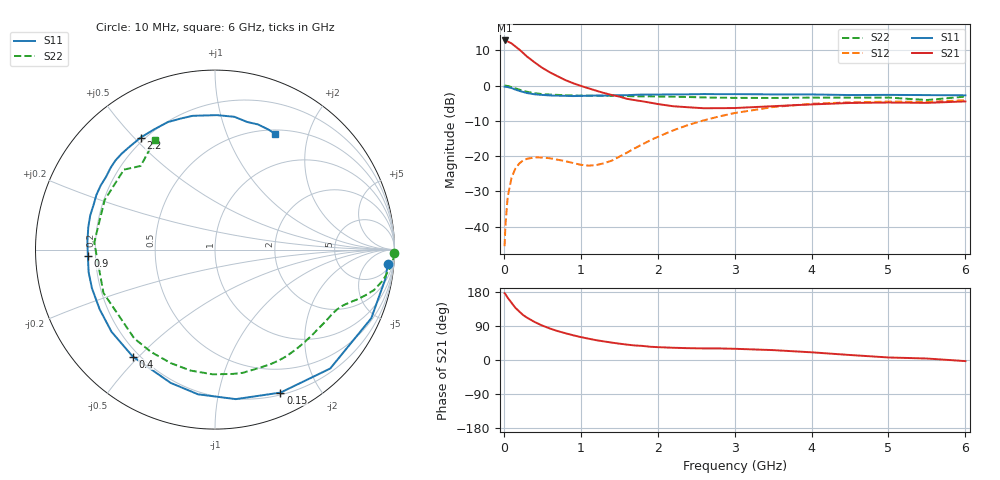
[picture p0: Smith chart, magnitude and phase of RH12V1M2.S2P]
! SIEMENS Small Signal Semiconductors
! BFR106
! Si NPN RF Bipolar Junction Transistor in SOT23
! VCE = 12 V  IC = 1.2 mA
! Common Emitter S-Parameters:  August  1996
# GHz  S  MA  R  50
!  f  S11  S21  S12  S22
! GHz  MAG  ANG  MAG  ANG  MAG  ANG  MAG  ANG
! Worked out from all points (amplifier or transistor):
!   36 points, 10 MHz to 6 GHz, reference 50 ohm
!   highest |S21| = 12.8 dB at 10 MHz (marker M1)
!   |S21| within 3 dB of that: start of sweep to 223.1 MHz
!   unconditionally stable (mu >= 1): 845.2 MHz to 1.802 GHz; 3.494 GHz to end of sweep
!   at 250 MHz: K = 0.27, MSG = 15.2 dB, |S12| = -21.2 dB
!   at 1.4 GHz: K = 1.34, MAG = 5.8 dB, |S12| = -21.3 dB
!   at 6 GHz: K = 1.02, MAG = -1.0 dB, |S12| = -4.2 dB
!   S11 on the Smith chart (normalised r, x): 10 MHz: 8, -20; 150 MHz: 0.22, -1.53; 400 MHz: 0.18, -0.48; 900 MHz: 0.17, -0.02; 2.2 GHz: 0.18, +0.52; 6 GHz: 0.55, +1.50
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0.01  0.9657 -4.9  4.352 176.2  0.0053 90.0  0.9999 -1.1
0.02  0.9637 -9.6  4.311 174.0  0.0102 83.5  0.9978 -2.3
0.05  0.951 -23.7  4.21 164.2  0.0265 76.6  0.9838 -5.5
0.1  0.9226 -45.9  3.959 151.0  0.0494 65.0  0.9514 -10.4
0.15  0.8763 -65.4  3.578 137.7  0.0666 54.5  0.914 -14.3
0.2  0.8411 -82.1  3.245 128.1  0.0785 46.9  0.8759 -16.9
0.25  0.8117 -96.7  2.9 118.7  0.0868 39.8  0.8417 -19.2
0.3  0.7826 -108.4  2.581 111.9  0.0916 35.5  0.8165 -20.7
0.4  0.7517 -127.5  2.129 100.3  0.0959 28.3  0.7787 -23.5
0.5  0.7363 -141.5  1.779 90.8  0.0956 23.8  0.7574 -26.1
0.6  0.7236 -152.6  1.535 83.0  0.0932 21.8  0.7446 -28.9
0.9  0.7092 -177.2  1.08 65.3  0.0799 27.0  0.7238 -38.1
1.1  0.717 170.0  0.914 56.3  0.0733 39.3  0.7179 -45.2
1.6  0.7298 146.3  0.648 40.6  0.1119 74.8  0.7093 -64.3
2.2  0.7493 123.6  0.509 32.3  0.2314 77.5  0.695 -91.1
2.8  0.7548 104.7  0.478 30.5  0.3652 64.5  0.6725 -122.1
3.5  0.7493 89.2  0.51 26.1  0.4958 46.0  0.6667 -158.8
4  0.7478 81.7  0.54 20.3  0.5516 33.0  0.6739 176.6
4.5  0.7333 75.8  0.566 13.2  0.5781 21.8  0.6741 155.8
5  0.7374 71.0  0.575 6.7  0.591 12.6  0.6752 138.7
5.5  0.732 65.9  0.568 3.9  0.588 8.1  0.6233 131.6
6  0.7265 62.7  0.596 -2.9  0.6188 -0.3  0.6971 118.8
